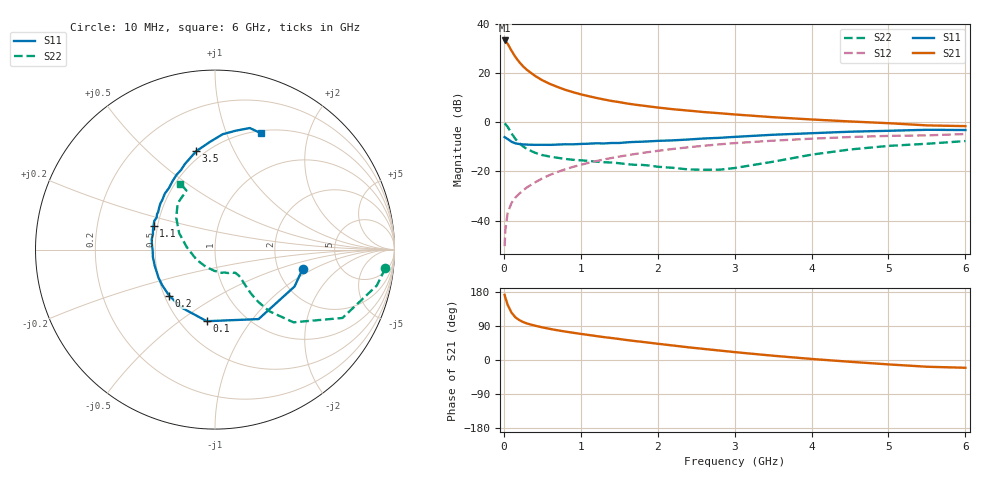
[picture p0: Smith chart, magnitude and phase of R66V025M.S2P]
! SIEMENS Small Signal Semiconductors
! BFR193
! Si NPN RF Bipolar Junction Transistor in SOT23
! VCE = 6 V  IC = 25 mA
! Common Emitter S-Parameters:  May  1996
# GHz  S  MA  R  50
!  f  S11  S21  S12  S22
! GHz  MAG  ANG  MAG  ANG  MAG  ANG  MAG  ANG
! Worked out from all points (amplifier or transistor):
!   36 points, 10 MHz to 6 GHz, reference 50 ohm
!   highest |S21| = 33.4 dB at 10 MHz (marker M1)
!   |S21| within 3 dB of that: start of sweep to 78.8 MHz
!   unconditionally stable (mu >= 1): 530.2 MHz to 2.014 GHz
!   at 250 MHz: K = 0.86, MSG = 25.3 dB, |S12| = -27.7 dB
!   at 1.4 GHz: K = 1.02, MAG = 10.7 dB, |S12| = -14.5 dB
!   at 6 GHz: K = 0.94, MSG = 1.6 dB, |S12| = -4.8 dB
!   S11 on the Smith chart (normalised r, x): 10 MHz: 2.74, -0.80; 100 MHz: 0.67, -0.64; 200 MHz: 0.53, -0.31; 1.1 GHz: 0.48, +0.15; 3.5 GHz: 0.45, +0.72; 6 GHz: 0.53, +1.33
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0.01  0.4999 -12.6  46.54 171.9  0.003 86.6  0.9543 -6.3
0.02  0.4886 -24.9  45.59 164.3  0.0065 79.9  0.9237 -12.5
0.05  0.457 -57.9  39.63 145.3  0.0144 71.4  0.806 -28.2
0.1  0.4016 -96.6  28.76 124.9  0.0228 64.9  0.5962 -42.8
0.15  0.373 -120.3  21.47 112.7  0.0293 63.5  0.4583 -48.6
0.2  0.3618 -135.0  16.94 105.5  0.0351 65.2  0.3764 -50.4
0.25  0.3549 -146.0  13.82 100.2  0.041 66.2  0.3223 -50.7
0.3  0.3516 -153.5  11.72 96.4  0.0472 67.9  0.287 -50.3
0.4  0.3477 -165.1  8.961 90.8  0.0591 69.2  0.2419 -49.1
0.5  0.3486 -173.1  7.195 86.1  0.0721 70.0  0.2153 -47.8
0.6  0.3474 -179.5  6.053 82.0  0.0851 69.9  0.2002 -47.5
0.8  0.3572 170.8  4.587 75.0  0.1108 69.2  0.1795 -48.3
1  0.3629 162.2  3.718 68.9  0.1361 67.6  0.1683 -50.1
1.1  0.367 158.8  3.417 66.1  0.1496 66.7  0.1639 -52.4
1.3  0.3711 151.2  2.922 60.4  0.1752 64.4  0.1541 -56.5
1.6  0.3909 142.5  2.42 52.6  0.2129 60.7  0.1407 -65.8
2.2  0.4291 126.6  1.849 38.2  0.2869 52.6  0.1183 -92.1
2.8  0.4829 113.0  1.534 25.1  0.3556 43.8  0.1084 -136.4
3.5  0.5583 100.8  1.271 11.3  0.423 33.0  0.1575 175.3
4.5  0.6442 86.2  1.042 -4.7  0.5014 18.9  0.2795 140.6
5.5  0.7047 74.0  0.866 -17.8  0.542 4.9  0.3658 115.8
6  0.6965 68.4  0.837 -20.5  0.5778 0.8  0.4155 117.7
